|   IBIS model for TI xxx DSP
[IBIS Ver]   5.1
[Disclaimer]   Please be aware that in the absence of a written agreement
|   Texas Instruments(TI) assumes no liability for:
|   (1) The accuracy of the IBIS models provided to your company,
|   however, the IBIS model is compliant to industry standard
|   IQ Level 2a.  Refer to IBIS Quality Section below for
|   for full details.
|   (2) The proper functioning of these Models in your design
|   or for any resulting applications
|   (3) Infringement of patents, copyrights or intellectual
|   property rights resulting from your use of these
|   models.
|   TI provides IBIS Models as a service to our customers and
|   therefore reserves the right to limit distribution of the
|   Models.  The information is subject to change without notice.
[File Name]  sprm812.ibs
[File Rev]   0.1
|   -Initial version
|   -Updated Package model
[Date]   28 July 2022
[Source]   Texas Instruments Incorporated
[Copyright]   Property of Texas Instruments Incorporated.
|   Unauthorized reproduction and/or distribution is strictly.
|   prohibited.
|   This product is protected under copyright law and trade
|   secret law as an unpublished work.
|   Created 2012,(C) Copyright 1999-2012,
|   Texas Instruments Incorporated., All Rights Reserved.
|   These commodities are under the U.S. Government
|   distribution license control. As such,they are not to be
|   re-exported without the prior approval of the U.S.
|   Department of Commerce.
[Notes]
   ADC pins are marked as NC
   Clock pins are marked as NC
   nReset pin marked as NC
   TEMP Sensor pins marked as NC
|   Revision History
|   GERNERAL COMMENT: All IBIS Quality Notes below reflect latest release
|   and version of IBIS File
|   File passes ibischk6.0 with 0 errors and 24 warnings
|   Component AM273
[Component] AM273
[Manufacturer] Texas Instruments
[Package Model] AM273_pkg
[Package]
|   typ   min   max
R_pkg   0.21352   0.10892   0.28767
L_pkg   3.868e-9   1.764e-9   5.903e-9
C_pkg   4.82e-13   3.248e-13   8.016e-13
[Pin]   Signal_name   model_name
M1   VBGAP   POWER
E4   VDD   POWER
E5   VDD   POWER
H4   VDD   POWER
H5   VDD   POWER
L4   VDD   POWER
L5   VDD   POWER
D7   VDD   POWER
M7   VDD   POWER
D9   VDD   POWER
M9   VDD   POWER
H11   VDD   POWER
L11   VDD   POWER
H12   VDD   POWER
L12   VDD   POWER
E11   VDD   POWER
E12   VDD   POWER
K14   VDD_SRAM1   POWER
G3   VDD_SRAM2   POWER
M6   VDD_SRAM3   POWER
F4   VIOIN   POWER
C10   VIOIN   POWER
N10   VIOIN   POWER
F13   VIOIN   POWER
K13   VIOIN   POWER
J4   VIOIN_18   POWER
C8   VIOIN_18   POWER
N8   VIOIN_18   POWER
J12   VIOIN_18   POWER
M2   VIOIN_18ADC   POWER
N2   VIOIN_18CLK   POWER
L13   VNWA   POWER
N7   VPP   POWER
L1   ADC1   NC
P3   ADC2   NC
K2   ADC3   NC
K1   ADC4   NC
J1   ADC5   NC
L2   ADC6   NC
N3   ADC7   NC
J2   ADC8   NC
M3   ADC9   NC
N1   CLKM   NC
P1   CLKP   NC
D2   MSS_EPWMA0   bc1833dv40dcpbfbp18ll_ssdlv
C13   MSS_EPWMA1   bc1833dv40dcpbfbp18ll_ssdlv
D15   MSS_EPWMA_SYNCI   bc1833dv40dcpbfbp18ll_ssdlv
D3   MSS_EPWMB0   bc1833dv40dcpbfbp18ll_ssdlv
D14   MSS_EPWMB1   bc1833dv40dcpbfbp18ll_ssdlv
E1   MSS_EPWMC0   bc1833dv40dcpbfbp18ll_ssdlv
D13   MSS_EPWMC1   bc1833dv40dcpbfbp18ll_ssdlv
F3   MSS_GPIO_0   bc1833dv40dcpbfbp18ll_ssdlv
F2   MSS_GPIO_1   bc1833dv40dcpbfbp18ll_ssdlv
F1   MSS_GPIO_2   bc1833dv40dcpbfbp18ll_ssdlv
E15   MSS_GPIO_7   bc1833dv40dcpbfbp18ll_ssdlv
B4   MSS_GPIO_8   bc1833dv40dcpbfbp18ll_ssdlv
E3   MSS_GPIO_14   bc1833dv40dcpbfbp18ll_ssdlv
E2   MSS_GPIO_28   bc1833dv40dcpbfbp18ll_ssdlv
C14   MSS_GPIO_29   bc1833dv40dcpbfbp18ll_ssdlv
A3   MSS_I2CA_SCL   bc1833dv40dcpbfbp18ll_ssdlv
A4   MSS_I2CA_SDA   bc1833dv40dcpbfbp18ll_ssdlv
B3   MSS_MCANA_RX   bc1833dv40dcpbfbp18ll_ssdlv
C3   MSS_MCANA_TX   bc1833dv40dcpbfbp18ll_ssdlv
M15   MSS_MDIO_CLK   bc1833dv40dcpbfbp18ll_ssdlv
M14   MSS_MDIO_DATA   bc1833dv40dcpbfbp18ll_ssdlv
B14   MSS_MIBSPIB_CLK   bc1833dv40dcpbfbp18ll_ssdlv
B15   MSS_MIBSPIB_CS0   bc1833dv40dcpbfbp18ll_ssdlv
C15   MSS_MIBSPIB_CS1   bc1833dv40dcpbfbp18ll_ssdlv
A14   MSS_MIBSPIB_MISO   bc1833dv40dcpbfbp18ll_ssdlv
B13   MSS_MIBSPIB_MOSI   bc1833dv40dcpbfbp18ll_ssdlv
B2   MSS_QSPI_0   bc1833dv40dcpbfbp18ll_ssdlv
A2   MSS_QSPI_1   bc1833dv40dcpbfbp18ll_ssdlv
C2   MSS_QSPI_2   bc1833dv40dcpbfbp18ll_ssdlv
B1   MSS_QSPI_3   bc1833dv40dcpbfbp18ll_ssdlv
D1   MSS_QSPI_CLK   bc1833dv40dcpbfbp18ll_ssdlv
C1   MSS_QSPI_CS   bc1833dv40dcpbfbp18ll_ssdlv
K15   MSS_RGMII_RCLK   bc1833dv40dcpbfbp18ll_ssdlv
G13   MSS_RGMII_RCTL   bc1833dv40dcpbfbp18ll_ssdlv
M13   MSS_RGMII_RD0   bc1833dv40dcpbfbp18ll_ssdlv
L15   MSS_RGMII_RD1   bc1833dv40dcpbfbp18ll_ssdlv
L14   MSS_RGMII_RD2   bc1833dv40dcpbfbp18ll_ssdlv
J13   MSS_RGMII_RD3   bc1833dv40dcpbfbp18ll_ssdlv
H15   MSS_RGMII_TCLK   bc1833dv40dcpbfbp18ll_ssdlv
G15   MSS_RGMII_TCTL   bc1833dv40dcpbfbp18ll_ssdlv
J14   MSS_RGMII_TD0   bc1833dv40dcpbfbp18ll_ssdlv
J15   MSS_RGMII_TD1   bc1833dv40dcpbfbp18ll_ssdlv
H13   MSS_RGMII_TD2   bc1833dv40dcpbfbp18ll_ssdlv
H14   MSS_RGMII_TD3   bc1833dv40dcpbfbp18ll_ssdlv
R3   MSS_UARTA_RX   bc1833dv40dcpbfbp18ll_ssdlh
R4   MSS_UARTA_TX   bc1833dv40dcpbfbp18ll_ssdlh
P4   MSS_UARTB_TX   bc1833dv40dcpbfbp18ll_ssdlh
H2   NERROR_IN   bc1833dv40dcpbfbp18ll_od_fs_ssdlv
H1   NERROR_OUT   bc1833dv40dcpbfbp18ll_od_fs_ssdlv
J3   NRESET   NC
R2   OSC_CLK_OUT_AUDIO   NC
E14   RCSS_ECAPA_CAPIN_PWMO   bc1833dv40dcpbfbp18ll_ssdlv
R14   RCSS_GPIO_39   bc1833dv40dcpbfbp18ll_ssdlv
R13   RCSS_I2CA_SCL   bc1833dv40dcpbfbp18ll_ssdlv
P13   RCSS_I2CA_SDA   bc1833dv40dcpbfbp18ll_ssdlv
B12   RCSS_MCASPA_ACLKR   bc1833dv40dcpbfbp18ll_ssdlh
A12   RCSS_MCASPA_ACLKX   bc1833dv40dcpbfbp18ll_ssdlh
A13   RCSS_MCASPA_AHCLKX   bc1833dv40dcpbfbp18ll_ssdlh
B11   RCSS_MCASPA_DAT0   bc1833dv40dcpbfbp18ll_ssdlh
C11   RCSS_MCASPA_DAT1   bc1833dv40dcpbfbp18ll_ssdlh
B7   RCSS_MCASPA_DAT2   bc1833dv40dcpbfbp18ll_ssdlh
C7   RCSS_MCASPA_DAT3   bc1833dv40dcpbfbp18ll_ssdlh
B6   RCSS_MCASPA_DAT4   bc1833dv40dcpbfbp18ll_ssdlh
A6   RCSS_MCASPA_DAT5   bc1833dv40dcpbfbp18ll_ssdlh
B5   RCSS_MCASPA_DAT6   bc1833dv40dcpbfbp18ll_ssdlh
A5   RCSS_MCASPA_DAT7   bc1833dv40dcpbfbp18ll_ssdlh
B10   RCSS_MCASPA_DAT8   bc1833dv40dcpbfbp18ll_ssdlh
A10   RCSS_MCASPA_DAT9   bc1833dv40dcpbfbp18ll_ssdlh
A9   RCSS_MCASPA_DAT10   bc1833dv40dcpbfbp18ll_ssdlh
C9   RCSS_MCASPA_DAT11   bc1833dv40dcpbfbp18ll_ssdlh
B9   RCSS_MCASPA_DAT12   bc1833dv40dcpbfbp18ll_ssdlh
A8   RCSS_MCASPA_DAT13   bc1833dv40dcpbfbp18ll_ssdlh
B8   RCSS_MCASPA_DAT14   bc1833dv40dcpbfbp18ll_ssdlh
A7   RCSS_MCASPA_DAT15   bc1833dv40dcpbfbp18ll_ssdlh
A11   RCSS_MCASPA_FSR   bc1833dv40dcpbfbp18ll_ssdlh
C12   RCSS_MCASPA_FSX   bc1833dv40dcpbfbp18ll_ssdlh
P7   RCSS_MCASPB_ACLKR   bc1833dv40dcpbfbp18ll_ssdlh
R8   RCSS_MCASPB_ACLKX   bc1833dv40dcpbfbp18ll_ssdlh
R7   RCSS_MCASPB_AHCLKX   bc1833dv40dcpbfbp18ll_ssdlh
R6   RCSS_MCASPB_DAT0   bc1833dv40dcpbfbp18ll_ssdlh
N5   RCSS_MCASPB_DAT1   bc1833dv40dcpbfbp18ll_ssdlh
P5   RCSS_MCASPB_DAT2   bc1833dv40dcpbfbp18ll_ssdlh
R5   RCSS_MCASPB_DAT3   bc1833dv40dcpbfbp18ll_ssdlh
N4   RCSS_MCASPB_DAT4   bc1833dv40dcpbfbp18ll_ssdlh
N6   RCSS_MCASPB_DAT5   bc1833dv40dcpbfbp18ll_ssdlh
P6   RCSS_MCASPB_FSR   bc1833dv40dcpbfbp18ll_ssdlh
P8   RCSS_MCASPB_FSX   bc1833dv40dcpbfbp18ll_ssdlh
R10   RCSS_MCASPC_ACLKR   bc1833dv40dcpbfbp18ll_ssdlh
R9   RCSS_MCASPC_ACLKX   bc1833dv40dcpbfbp18ll_ssdlh
P9   RCSS_MCASPC_AHCLKX   bc1833dv40dcpbfbp18ll_ssdlh
R11   RCSS_MCASPC_DAT0   bc1833dv40dcpbfbp18ll_ssdlh
P11   RCSS_MCASPC_DAT1   bc1833dv40dcpbfbp18ll_ssdlh
N11   RCSS_MCASPC_DAT2   bc1833dv40dcpbfbp18ll_ssdlh
R12   RCSS_MCASPC_DAT3   bc1833dv40dcpbfbp18ll_ssdlh
P12   RCSS_MCASPC_DAT4   bc1833dv40dcpbfbp18ll_ssdlh
N12   RCSS_MCASPC_DAT5   bc1833dv40dcpbfbp18ll_ssdlh
P10   RCSS_MCASPC_FSR   bc1833dv40dcpbfbp18ll_ssdlh
N9   RCSS_MCASPC_FSX   bc1833dv40dcpbfbp18ll_ssdlh
P15   RCSS_MIBSPIA_CLK   bc1833dv40dcpbfbp18ll_ssdlv
P14   RCSS_MIBSPIA_CS0   bc1833dv40dcpbfbp18ll_ssdlv
N13   RCSS_MIBSPIA_CS1   bc1833dv40dcpbfbp18ll_ssdlv
N14   RCSS_MIBSPIA_MISO   bc1833dv40dcpbfbp18ll_ssdlv
N15   RCSS_MIBSPIA_MOSI   bc1833dv40dcpbfbp18ll_ssdlv
E13   RCSS_UARTA_CTS   bc1833dv40dcpbfbp18ll_ssdlv
F15   RCSS_UARTA_RTS   bc1833dv40dcpbfbp18ll_ssdlv
G14   RCSS_UARTA_RX   bc1833dv40dcpbfbp18ll_ssdlv
F14   RCSS_UARTA_TX   bc1833dv40dcpbfbp18ll_ssdlv
D4   TCK   bc1833dv40dcpbfbp18ll_ssdlh
C5   TDI   bc1833dv40dcpbfbp18ll_ssdlh
C6   TDO   bc1833dv40dcpbfbp18ll_ssdlh
L3   TEMP_SENSOR_1   NC
K3   TEMP_SENSOR_2   NC
C4   TMS   bc1833dv40dcpbfbp18ll_ssdlh
H3   WARM_RESET   bc1833dv40dcpbfbp18ll_od_fs_ssdlv
G1   XREF_CLK0   NC
G2   XREF_CLK1   NC
R1   VSS   GND
P2   VSS   GND
A1   VSS   GND
D5   VSS   GND
D6   VSS   GND
G4   VSS   GND
K4   VSS   GND
M8   VSS   GND
D11   VSS   GND
D12   VSS   GND
F5   VSS   GND
G5   VSS   GND
K5   VSS   GND
J5   VSS   GND
E6   VSS   GND
F6   VSS   GND
H6   VSS   GND
G6   VSS   GND
K6   VSS   GND
J6   VSS   GND
L6   VSS   GND
E7   VSS   GND
E8   VSS   GND
D8   VSS   GND
F7   VSS   GND
F8   VSS   GND
H7   VSS   GND
G7   VSS   GND
H8   VSS   GND
G8   VSS   GND
K7   VSS   GND
J7   VSS   GND
K8   VSS   GND
J8   VSS   GND
L7   VSS   GND
L8   VSS   GND
E9   VSS   GND
E10   VSS   GND
D10   VSS   GND
F9   VSS   GND
F10   VSS   GND
H9   VSS   GND
G9   VSS   GND
H10   VSS   GND
G10   VSS   GND
K9   VSS   GND
J9   VSS   GND
K10   VSS   GND
J10   VSS   GND
L9   VSS   GND
L10   VSS   GND
M10   VSS   GND
F11   VSS   GND
G11   VSS   GND
K11   VSS   GND
J11   VSS   GND
M11   VSS   GND
F12   VSS   GND
G12   VSS   GND
M12   VSS   GND
M5   VSS   GND
M4   VSS   GND
K12   VSS   GND
R15   VSS   GND
A15   VSS   GND
|   BC1833DV40DCPBFBP18LL_SSDLH
[Model Selector] bc1833dv40dcpbfbp18ll_ssdlh
|SC1 IS A SLEW RATE CONTROL PIN
|5% SUPPLY VARIATION MODES WITH 1.8V NOM SUPPLY
BC40D_H_PUPDOFF_5P_SC1_1P8  Cell operated at 1.8(nom)
|BC40D_H_PUPDOFF_5P_SC1_1P8; BUFFER WITH WEAK PULUP/PULLDOWN OFF AT 5% SUPPLY
|VARIATION WITH SC1=1 MEANING SLOW MODE OF OPERATION
BC40D_H_PD_ON_5P_!SC1_1P8  Cell operated at 1.8(nom)
|BC40D_H_PD_ON_5P_!SC1_1P8; BUFFER WITH WEAK_PULLDOWN_ON AT 5% SUPPLY
|VARIATION WITH SC1=0 MEANING FAST MODE OF OPERATION
BC40D_H_PD_ON_5P_SC1_1P8  Cell operated at 1.8(nom)
|BC40D_H_PD_ON_5P_SC1_1P8; BUFFER WITH WEAK_PULLDOWN_ON AT 5% SUPPLY
|VARIATION WITH SC1=1 MEANING SLOW MODE OF OPERATION
BC40D_H_PU_ON_5P_!SC1_1P8  Cell operated at 1.8(nom)
|BC40D_H_PU_ON_5P_!SC1_1P8; BUFFER WITH WEAK_PULLUP_ON AT 5% SUPPLY
|VARIATION WITH SC1=0 MEANING FAST MODE OF OPERATION
BC40D_H_PUPDOFF_5P_!SC1_1P8  Cell operated at 1.8(nom)
|BC40D_H_PUPDOFF_5P_!SC1_1P8; BUFFER WITH WEAK PULUP/PULLDOWN OFF AT 5% SUPPLY
|VARIATION WITH SC1=0 MEANING FAST MODE OF OPERATION
BC40D_H_PU_ON_5P_SC1_1P8  Cell operated at 1.8(nom)
|BC40D_H_PU_ON_5P_SC1_1P8; BUFFER WITH WEAK_PULLUP_ON AT 5% SUPPLY
|VARIATION WITH SC1=1 MEANING SLOW MODE OF OPERATION
|5% SUPPLY VARIATION MODES WITH 3.3V NOM SUPPLY
BC40D_H_PUPDOFF_5P_SC1_3P3  Cell operated at 3.3(nom)
|BC40D_H_PUPDOFF_5P_SC1_3P3; BUFFER WITH WEAK PULUP/PULLDOWN OFF AT 5% SUPPLY
|VARIATION WITH SC1=1 MEANING SLOW MODE OF OPERATION
BC40D_H_PD_ON_5P_!SC1_3P3  Cell operated at 3.3(nom)
|BC40D_H_PD_ON_5P_!SC1_3P3; BUFFER WITH WEAK_PULLDOWN_ON AT 5% SUPPLY
|VARIATION WITH SC1=0 MEANING FAST MODE OF OPERATION
BC40D_H_PD_ON_5P_SC1_3P3  Cell operated at 3.3(nom)
|BC40D_H_PD_ON_5P_SC1_3P3; BUFFER WITH WEAK_PULLDOWN_ON AT 5% SUPPLY
|VARIATION WITH SC1=1 MEANING SLOW MODE OF OPERATION
BC40D_H_PU_ON_5P_!SC1_3P3  Cell operated at 3.3(nom)
|BC40D_H_PU_ON_5P_!SC1_3P3; BUFFER WITH WEAK_PULLUP_ON AT 5% SUPPLY
|VARIATION WITH SC1=0 MEANING FAST MODE OF OPERATION
BC40D_H_PUPDOFF_5P_!SC1_3P3  Cell operated at 3.3(nom)
|BC40D_H_PUPDOFF_5P_!SC1_3P3; BUFFER WITH WEAK PULUP/PULLDOWN OFF AT 5% SUPPLY
|VARIATION WITH SC1=0 MEANING FAST MODE OF OPERATION
BC40D_H_PU_ON_5P_SC1_3P3  Cell operated at 3.3(nom)
|BC40D_H_PU_ON_5P_SC1_3P3; BUFFER WITH WEAK_PULLUP_ON AT 5% SUPPLY
|VARIATION WITH SC1=1 MEANING SLOW MODE OF OPERATION
| 10% SUPPLY VARIATION MODES WITH 1.8V NOM SUPPLY
BC40D_H_PUPDOFF_10P_SC1_1P8  Cell operated at 1.8(nom)
|BC40D_H_PUPDOFF_10P_SC1_1P8; BUFFER WITH WEAK PULUP/PULLDOWN OFF AT 10% SUPPLY
|VARIATION WITH SC1=1 MEANING SLOW MODE OF OPERATION
BC40D_H_PD_ON_10P_!SC1_1P8  Cell operated at 1.8(nom)
|BC40D_H_PD_ON_10P_!SC1_1P8; BUFFER WITH WEAK_PULLDOWN_ON AT 10% SUPPLY
|VARIATION WITH SC1=0 MEANING FAST MODE OF OPERATION
BC40D_H_PD_ON_10P_SC1_1P8  Cell operated at 1.8(nom)
|BC40D_H_PD_ON_10P_SC1_1P8; BUFFER WITH WEAK_PULLDOWN_ON AT 10% SUPPLY
|VARIATION WITH SC1=1 MEANING SLOW MODE OF OPERATION
BC40D_H_PU_ON_10P_!SC1_1P8  Cell operated at 1.8(nom)
|BC40D_H_PU_ON_10P_!SC1_1P8; BUFFER WITH WEAK_PULLUP_ON AT 10% SUPPLY
|VARIATION WITH SC1=0 MEANING FAST MODE OF OPERATION
BC40D_H_PUPDOFF_10P_!SC1_1P8  Cell operated at 1.8(nom)
|BC40D_H_PUPDOFF_10P_!SC1_1P8; BUFFER WITH WEAK PULUP/PULLDOWN OFF AT 10% SUPPLY
|VARIATION WITH SC1=0 MEANING FAST MODE OF OPERATION
BC40D_H_PU_ON_10P_SC1_1P8  Cell operated at 1.8(nom)
|BC40D_H_PU_ON_10P_SC1_1P8; BUFFER WITH WEAK_PULLUP_ON AT 10% SUPPLY
|VARIATION WITH SC1=1 MEANING SLOW MODE OF OPERATION
| 10% SUPPLY VARIATION MODES WITH 3.3V NOM SUPPLY
BC40D_H_PUPDOFF_10P_SC1_3P3  Cell operated at 3.3(nom)
|BC40D_H_PUPDOFF_10P_SC1_3P3; BUFFER WITH WEAK PULUP/PULLDOWN OFF AT 10% SUPPLY
|VARIATION WITH SC1=1 MEANING SLOW MODE OF OPERATION
BC40D_H_PD_ON_10P_!SC1_3P3  Cell operated at 3.3(nom)
|BC40D_H_PD_ON_10P_!SC1_3P3; BUFFER WITH WEAK_PULLDOWN_ON 10% SUPPLY
|VARIATION WITH SC1=0 MEANING FAST MODE OF OPERATION
BC40D_H_PD_ON_10P_SC1_3P3  Cell operated at 3.3(nom)
|BC40D_H_PD_ON_10P_SC1_3P3; BUFFER WITH WEAK_PULLDOWN_ON AT 10% SUPPLY
|VARIATION WITH SC1=1 MEANING SLOW MODE OF OPERATION
BC40D_H_PU_ON_10P_!SC1_3P3  Cell operated at 3.3(nom)
|BC40D_H_PU_ON_10P_!SC1_3P3; BUFFER WITH WEAK_PULLUP_ON AT 10% SUPPLY
|VARIATION WITH SC1=0 MEANING FAST MODE OF OPERATION
BC40D_H_PUPDOFF_10P_!SC1_3P3  Cell operated at 3.3(nom)
|BC40D_H_PUPDOFF_10P_!SC1_3P3; BUFFER WITH WEAK PULUP/PULLDOWN OFF AT 10% SUPPLY
|VARIATION WITH SC1=0 MEANING FAST MODE OF OPERATION
BC40D_H_PU_ON_10P_SC1_3P3  Cell operated at 3.3(nom)
|BC40D_H_PU_ON_10P_SC1_3P3; BUFFER WITH WEAK_PULLUP_ON AT 10% SUPPLY
|VARIATION WITH SC1=1 MEANING SLOW MODE OF OPERATION
|   BC1833DV40DCPBFBP18LL_SSDLV
[Model Selector] bc1833dv40dcpbfbp18ll_ssdlv
|SC1 IS A SLEW RATE CONTROL PIN
|5% SUPPLY VARIATION MODES WITH 1.8V NOM SUPPLY
BC40D_V_PUPDOFF_5P_SC1_1P8  Cell operated at 1.8(nom)
|BC40D_V_PUPDOFF_5P_SC1_1P8; BUFFER WITH WEAK PULUP/PULLDOWN OFF AT 5% SUPPLY
|VARIATION WITH SC1=1 MEANING SLOW MODE OF OPERATION
BC40D_V_PD_ON_5P_!SC1_1P8  Cell operated at 1.8(nom)
|BC40D_V_PD_ON_5P_!SC1_1P8; BUFFER WITH WEAK_PULLDOWN_ON AT 5% SUPPLY
|VARIATION WITH SC1=0 MEANING FAST MODE OF OPERATION
BC40D_V_PD_ON_5P_SC1_1P8  Cell operated at 1.8(nom)
|BC40D_V_PD_ON_5P_SC1_1P8; BUFFER WITH WEAK_PULLDOWN_ON AT 5% SUPPLY
|VARIATION WITH SC1=1 MEANING SLOW MODE OF OPERATION
BC40D_V_PU_ON_5P_!SC1_1P8  Cell operated at 1.8(nom)
|BC40D_V_PU_ON_5P_!SC1_1P8; BUFFER WITH WEAK_PULLUP_ON AT 5% SUPPLY
|VARIATION WITH SC1=0 MEANING FAST MODE OF OPERATION
BC40D_V_PUPDOFF_5P_!SC1_1P8  Cell operated at 1.8(nom)
|BC40D_V_PUPDOFF_5P_!SC1_1P8; BUFFER WITH WEAK PULUP/PULLDOWN OFF AT 5% SUPPLY
|VARIATION WITH SC1=0 MEANING FAST MODE OF OPERATION
BC40D_V_PU_ON_5P_SC1_1P8  Cell operated at 1.8(nom)
|BC40D_V_PU_ON_5P_SC1_1P8; BUFFER WITH WEAK_PULLUP_ON AT 5% SUPPLY
|VARIATION WITH SC1=1 MEANING SLOW MODE OF OPERATION
|5% SUPPLY VARIATION MODES WITH 3.3V NOM SUPPLY
BC40D_V_PUPDOFF_5P_SC1_3P3  Cell operated at 3.3(nom)
|BC40D_V_PUPDOFF_5P_SC1_3P3; BUFFER WITH WEAK PULUP/PULLDOWN OFF AT 5% SUPPLY
|VARIATION WITH SC1=1 MEANING SLOW MODE OF OPERATION
BC40D_V_PD_ON_5P_!SC1_3P3  Cell operated at 3.3(nom)
|BC40D_V_PD_ON_5P_!SC1_3P3; BUFFER WITH WEAK_PULLDOWN_ON AT 5% SUPPLY
|VARIATION WITH SC1=0 MEANING FAST MODE OF OPERATION
BC40D_V_PD_ON_5P_SC1_3P3  Cell operated at 3.3(nom)
|BC40D_V_PD_ON_5P_SC1_3P3; BUFFER WITH WEAK_PULLDOWN_ON AT 5% SUPPLY
|VARIATION WITH SC1=1 MEANING SLOW MODE OF OPERATION
BC40D_V_PU_ON_5P_!SC1_3P3  Cell operated at 3.3(nom)
|BC40D_V_PU_ON_5P_!SC1_3P3; BUFFER WITH WEAK_PULLUP_ON AT 5% SUPPLY
|VARIATION WITH SC1=0 MEANING FAST MODE OF OPERATION
BC40D_V_PUPDOFF_5P_!SC1_3P3  Cell operated at 3.3(nom)
|BC40D_V_PUPDOFF_5P_!SC1_3P3; BUFFER WITH WEAK PULUP/PULLDOWN OFF AT 5% SUPPLY
|VARIATION WITH SC1=0 MEANING FAST MODE OF OPERATION
BC40D_V_PU_ON_5P_SC1_3P3  Cell operated at 3.3(nom)
|BC40D_V_PU_ON_5P_SC1_3P3; BUFFER WITH WEAK_PULLUP_ON AT 5% SUPPLY
|VARIATION WITH SC1=1 MEANING SLOW MODE OF OPERATION
| 10% SUPPLY VARIATION MODES WITH 1.8V NOM SUPPLY
BC40D_V_PUPDOFF_10P_SC1_1P8  Cell operated at 1.8(nom)
|BC40D_V_PUPDOFF_10P_SC1_1P8; BUFFER WITH WEAK PULUP/PULLDOWN OFF AT 10% SUPPLY
|VARIATION WITH SC1=1 MEANING SLOW MODE OF OPERATION
BC40D_V_PD_ON_10P_!SC1_1P8  Cell operated at 1.8(nom)
|BC40D_V_PD_ON_10P_!SC1_1P8; BUFFER WITH WEAK_PULLDOWN_ON AT 10% SUPPLY
|VARIATION WITH SC1=0 MEANING FAST MODE OF OPERATION
BC40D_V_PD_ON_10P_SC1_1P8  Cell operated at 1.8(nom)
|BC40D_V_PD_ON_10P_SC1_1P8; BUFFER WITH WEAK_PULLDOWN_ON AT 10% SUPPLY
|VARIATION WITH SC1=1 MEANING SLOW MODE OF OPERATION
BC40D_V_PU_ON_10P_!SC1_1P8  Cell operated at 1.8(nom)
|BC40D_V_PU_ON_10P_!SC1_1P8; BUFFER WITH WEAK_PULLUP_ON AT 10% SUPPLY
|VARIATION WITH SC1=0 MEANING FAST MODE OF OPERATION
BC40D_V_PUPDOFF_10P_!SC1_1P8  Cell operated at 1.8(nom)
|BC40D_V_PUPDOFF_10P_!SC1_1P8; BUFFER WITH WEAK PULUP/PULLDOWN OFF AT 10% SUPPLY
|VARIATION WITH SC1=0 MEANING FAST MODE OF OPERATION
BC40D_V_PU_ON_10P_SC1_1P8  Cell operated at 1.8(nom)
|BC40D_V_PU_ON_10P_SC1_1P8; BUFFER WITH WEAK_PULLUP_ON AT 10% SUPPLY
|VARIATION WITH SC1=1 MEANING SLOW MODE OF OPERATION
| 10% SUPPLY VARIATION MODES WITH 3.3V NOM SUPPLY
BC40D_V_PUPDOFF_10P_SC1_3P3  Cell operated at 3.3(nom)
|BC40D_V_PUPDOFF_10P_SC1_3P3; BUFFER WITH WEAK PULUP/PULLDOWN OFF AT 10% SUPPLY
|VARIATION WITH SC1=1 MEANING SLOW MODE OF OPERATION
BC40D_V_PD_ON_10P_!SC1_3P3  Cell operated at 3.3(nom)
|BC40D_V_PD_ON_10P_!SC1_3P3; BUFFER WITH WEAK_PULLDOWN_ON 10% SUPPLY
|VARIATION WITH SC1=0 MEANING FAST MODE OF OPERATION
BC40D_V_PD_ON_10P_SC1_3P3  Cell operated at 3.3(nom)
|BC40D_V_PD_ON_10P_SC1_3P3; BUFFER WITH WEAK_PULLDOWN_ON AT 10% SUPPLY
|VARIATION WITH SC1=1 MEANING SLOW MODE OF OPERATION
BC40D_V_PU_ON_10P_!SC1_3P3  Cell operated at 3.3(nom)
|BC40D_V_PU_ON_10P_!SC1_3P3; BUFFER WITH WEAK_PULLUP_ON AT 10% SUPPLY
|VARIATION WITH SC1=0 MEANING FAST MODE OF OPERATION
BC40D_V_PUPDOFF_10P_!SC1_3P3  Cell operated at 3.3(nom)
|BC40D_V_PUPDOFF_10P_!SC1_3P3; BUFFER WITH WEAK PULUP/PULLDOWN OFF AT 10% SUPPLY
|VARIATION WITH SC1=0 MEANING FAST MODE OF OPERATION
BC40D_V_PU_ON_10P_SC1_3P3  Cell operated at 3.3(nom)
|BC40D_V_PU_ON_10P_SC1_3P3; BUFFER WITH WEAK_PULLUP_ON AT 10% SUPPLY
|VARIATION WITH SC1=1 MEANING SLOW MODE OF OPERATION
|   BC1833DV40DCPBFBP18LL_OD_FS_SSDLV
[Model Selector] bc1833dv40dcpbfbp18ll_od_fs_ssdlv
|SC1 IS A SLEW RATE CONTROL PIN
|5% SUPPLY VARIATION MODES WITH 1.8V NOM SUPPLY
BC40D_V_PUPDOFF_5P_SC1_1P8  Cell operated at 1.8(nom)
|BC40D_V_PUPDOFF_5P_SC1_1P8; BUFFER WITH WEAK PULUP/PULLDOWN OFF AT 5% SUPPLY
|VARIATION WITH SC1=1 MEANING SLOW MODE OF OPERATION
BC40D_V_PD_ON_5P_!SC1_1P8  Cell operated at 1.8(nom)
|BC40D_V_PD_ON_5P_!SC1_1P8; BUFFER WITH WEAK_PULLDOWN_ON AT 5% SUPPLY
|VARIATION WITH SC1=0 MEANING FAST MODE OF OPERATION
BC40D_V_PD_ON_5P_SC1_1P8  Cell operated at 1.8(nom)
|BC40D_V_PD_ON_5P_SC1_1P8; BUFFER WITH WEAK_PULLDOWN_ON AT 5% SUPPLY
|VARIATION WITH SC1=1 MEANING SLOW MODE OF OPERATION
BC40D_V_PU_ON_5P_!SC1_1P8  Cell operated at 1.8(nom)
|BC40D_V_PU_ON_5P_!SC1_1P8; BUFFER WITH WEAK_PULLUP_ON AT 5% SUPPLY
|VARIATION WITH SC1=0 MEANING FAST MODE OF OPERATION
BC40D_V_PUPDOFF_5P_!SC1_1P8  Cell operated at 1.8(nom)
|BC40D_V_PUPDOFF_5P_!SC1_1P8; BUFFER WITH WEAK PULUP/PULLDOWN OFF AT 5% SUPPLY
|VARIATION WITH SC1=0 MEANING FAST MODE OF OPERATION
BC40D_V_PU_ON_5P_SC1_1P8  Cell operated at 1.8(nom)
|BC40D_V_PU_ON_5P_SC1_1P8; BUFFER WITH WEAK_PULLUP_ON AT 5% SUPPLY
|VARIATION WITH SC1=1 MEANING SLOW MODE OF OPERATION
|5% SUPPLY VARIATION MODES WITH 3.3V NOM SUPPLY
BC40D_V_PUPDOFF_5P_SC1_3P3  Cell operated at 3.3(nom)
|BC40D_V_PUPDOFF_5P_SC1_3P3; BUFFER WITH WEAK PULUP/PULLDOWN OFF AT 5% SUPPLY
|VARIATION WITH SC1=1 MEANING SLOW MODE OF OPERATION
BC40D_V_PD_ON_5P_!SC1_3P3  Cell operated at 3.3(nom)
|BC40D_V_PD_ON_5P_!SC1_3P3; BUFFER WITH WEAK_PULLDOWN_ON AT 5% SUPPLY
|VARIATION WITH SC1=0 MEANING FAST MODE OF OPERATION
BC40D_V_PD_ON_5P_SC1_3P3  Cell operated at 3.3(nom)
|BC40D_V_PD_ON_5P_SC1_3P3; BUFFER WITH WEAK_PULLDOWN_ON AT 5% SUPPLY
|VARIATION WITH SC1=1 MEANING SLOW MODE OF OPERATION
BC40D_V_PU_ON_5P_!SC1_3P3  Cell operated at 3.3(nom)
|BC40D_V_PU_ON_5P_!SC1_3P3; BUFFER WITH WEAK_PULLUP_ON AT 5% SUPPLY
|VARIATION WITH SC1=0 MEANING FAST MODE OF OPERATION
BC40D_V_PUPDOFF_5P_!SC1_3P3  Cell operated at 3.3(nom)
|BC40D_V_PUPDOFF_5P_!SC1_3P3; BUFFER WITH WEAK PULUP/PULLDOWN OFF AT 5% SUPPLY
|VARIATION WITH SC1=0 MEANING FAST MODE OF OPERATION
BC40D_V_PU_ON_5P_SC1_3P3  Cell operated at 3.3(nom)
|BC40D_V_PU_ON_5P_SC1_3P3; BUFFER WITH WEAK_PULLUP_ON AT 5% SUPPLY
|VARIATION WITH SC1=1 MEANING SLOW MODE OF OPERATION
| 10% SUPPLY VARIATION MODES WITH 1.8V NOM SUPPLY
BC40D_V_PUPDOFF_10P_SC1_1P8  Cell operated at 1.8(nom)
|BC40D_V_PUPDOFF_10P_SC1_1P8; BUFFER WITH WEAK PULUP/PULLDOWN OFF AT 10% SUPPLY
|VARIATION WITH SC1=1 MEANING SLOW MODE OF OPERATION
BC40D_V_PD_ON_10P_!SC1_1P8  Cell operated at 1.8(nom)
|BC40D_V_PD_ON_10P_!SC1_1P8; BUFFER WITH WEAK_PULLDOWN_ON AT 10% SUPPLY
|VARIATION WITH SC1=0 MEANING FAST MODE OF OPERATION
BC40D_V_PD_ON_10P_SC1_1P8  Cell operated at 1.8(nom)
|BC40D_V_PD_ON_10P_SC1_1P8; BUFFER WITH WEAK_PULLDOWN_ON AT 10% SUPPLY
|VARIATION WITH SC1=1 MEANING SLOW MODE OF OPERATION
BC40D_V_PU_ON_10P_!SC1_1P8  Cell operated at 1.8(nom)
|BC40D_V_PU_ON_10P_!SC1_1P8; BUFFER WITH WEAK_PULLUP_ON AT 10% SUPPLY
|VARIATION WITH SC1=0 MEANING FAST MODE OF OPERATION
BC40D_V_PUPDOFF_10P_!SC1_1P8  Cell operated at 1.8(nom)
|BC40D_V_PUPDOFF_10P_!SC1_1P8; BUFFER WITH WEAK PULUP/PULLDOWN OFF AT 10% SUPPLY
|VARIATION WITH SC1=0 MEANING FAST MODE OF OPERATION
BC40D_V_PU_ON_10P_SC1_1P8  Cell operated at 1.8(nom)
|BC40D_V_PU_ON_10P_SC1_1P8; BUFFER WITH WEAK_PULLUP_ON AT 10% SUPPLY
|VARIATION WITH SC1=1 MEANING SLOW MODE OF OPERATION
| 10% SUPPLY VARIATION MODES WITH 3.3V NOM SUPPLY
BC40D_V_PUPDOFF_10P_SC1_3P3  Cell operated at 3.3(nom)
|BC40D_V_PUPDOFF_10P_SC1_3P3; BUFFER WITH WEAK PULUP/PULLDOWN OFF AT 10% SUPPLY
|VARIATION WITH SC1=1 MEANING SLOW MODE OF OPERATION
BC40D_V_PD_ON_10P_!SC1_3P3  Cell operated at 3.3(nom)
|BC40D_V_PD_ON_10P_!SC1_3P3; BUFFER WITH WEAK_PULLDOWN_ON 10% SUPPLY
|VARIATION WITH SC1=0 MEANING FAST MODE OF OPERATION
BC40D_V_PD_ON_10P_SC1_3P3  Cell operated at 3.3(nom)
|BC40D_V_PD_ON_10P_SC1_3P3; BUFFER WITH WEAK_PULLDOWN_ON AT 10% SUPPLY
|VARIATION WITH SC1=1 MEANING SLOW MODE OF OPERATION
BC40D_V_PU_ON_10P_!SC1_3P3  Cell operated at 3.3(nom)
|BC40D_V_PU_ON_10P_!SC1_3P3; BUFFER WITH WEAK_PULLUP_ON AT 10% SUPPLY
|VARIATION WITH SC1=0 MEANING FAST MODE OF OPERATION
BC40D_V_PUPDOFF_10P_!SC1_3P3  Cell operated at 3.3(nom)
|BC40D_V_PUPDOFF_10P_!SC1_3P3; BUFFER WITH WEAK PULUP/PULLDOWN OFF AT 10% SUPPLY
|VARIATION WITH SC1=0 MEANING FAST MODE OF OPERATION
BC40D_V_PU_ON_10P_SC1_3P3  Cell operated at 3.3(nom)
|   Package Model
[Define Package Model]   AM273_pkg
[Manufacturer]   name 1
[OEM]   name 2
[Description]   138-pin Package
|[Number of Sections]   1
[Number of Pins]   138
[Pin Numbers]
|[Pin Name]  Net Number   Net Name   Net's All Pins
M1   | 1   VBGAP   M1
E4   | 2   VDD   E4
   |E5
   |H4
   |H5
   |L4
   |L5
   |D7
   |M7
   |D9
   |M9
   |H11
   |L11
   |H12
   |L12
   |E11
   |E12
K14   | 3   VDD_SRAM1   K14
G3   | 4   VDD_SRAM2   G3
M6   | 5   VDD_SRAM3   M6
F4   | 6   VIOIN   F4
   |C10
   |N10
   |F13
   |K13
J4   | 7   VIOIN_18   J4
   |C8
   |N8
   |J12
M2   | 8   VIOIN_18ADC   M2
N2   | 9   VIOIN_18CLK   N2
L13   | 10   VNWA   L13
N7   | 11   VPP   N7
L1   | 12   ADC1   L1
P3   | 13   ADC2   P3
K2   | 14   ADC3   K2
K1   | 15   ADC4   K1
J1   | 16   ADC5   J1
L2   | 17   ADC6   L2
N3   | 18   ADC7   N3
J2   | 19   ADC8   J2
M3   | 20   ADC9   M3
N1   | 21   CLKM   N1
P1   | 22   CLKP   P1
D2   | 23   MSS_EPWMA0   D2
C13   | 24   MSS_EPWMA1   C13
D15   | 25   MSS_EPWMA_SYNCI   D15
D3   | 26   MSS_EPWMB0   D3
D14   | 27   MSS_EPWMB1   D14
E1   | 28   MSS_EPWMC0   E1
D13   | 29   MSS_EPWMC1   D13
F3   | 30   MSS_GPIO_0   F3
F2   | 31   MSS_GPIO_1   F2
F1   | 32   MSS_GPIO_2   F1
E15   | 33   MSS_GPIO_7   E15
B4   | 34   MSS_GPIO_8   B4
E3   | 35   MSS_GPIO_14   E3
E2   | 36   MSS_GPIO_28   E2
C14   | 37   MSS_GPIO_29   C14
A3   | 38   MSS_I2CA_SCL   A3
A4   | 39   MSS_I2CA_SDA   A4
B3   | 40   MSS_MCANA_RX   B3
C3   | 41   MSS_MCANA_TX   C3
M15   | 42   MSS_MDIO_CLK   M15
M14   | 43   MSS_MDIO_DATA   M14
B14   | 44   MSS_MIBSPIB_CLK   B14
B15   | 45   MSS_MIBSPIB_CS0   B15
C15   | 46   MSS_MIBSPIB_CS1   C15
A14   | 47   MSS_MIBSPIB_MISO   A14
B13   | 48   MSS_MIBSPIB_MOSI   B13
B2   | 49   MSS_QSPI_0   B2
A2   | 50   MSS_QSPI_1   A2
C2   | 51   MSS_QSPI_2   C2
B1   | 52   MSS_QSPI_3   B1
D1   | 53   MSS_QSPI_CLK   D1
C1   | 54   MSS_QSPI_CS   C1
K15   | 55   MSS_RGMII_RCLK   K15
G13   | 56   MSS_RGMII_RCTL   G13
M13   | 57   MSS_RGMII_RD0   M13
L15   | 58   MSS_RGMII_RD1   L15
L14   | 59   MSS_RGMII_RD2   L14
J13   | 60   MSS_RGMII_RD3   J13
H15   | 61   MSS_RGMII_TCLK   H15
G15   | 62   MSS_RGMII_TCTL   G15
J14   | 63   MSS_RGMII_TD0   J14
J15   | 64   MSS_RGMII_TD1   J15
H13   | 65   MSS_RGMII_TD2   H13
H14   | 66   MSS_RGMII_TD3   H14
R3   | 67   MSS_UARTA_RX   R3
R4   | 68   MSS_UARTA_TX   R4
P4   | 69   MSS_UARTB_TX   P4
H2   | 70   NERROR_IN   H2
H1   | 71   NERROR_OUT   H1
J3   | 72   NRESET   J3
R2   | 73   OSC_CLK_OUT_AUDIO   R2
E14   | 74   RCSS_ECAPA_CAPIN_PWMO   E14
R14   | 75   RCSS_GPIO_39   R14
R13   | 76   RCSS_I2CA_SCL   R13
P13   | 77   RCSS_I2CA_SDA   P13
B12   | 78   RCSS_MCASPA_ACLKR   B12
A12   | 79   RCSS_MCASPA_ACLKX   A12
A13   | 80   RCSS_MCASPA_AHCLKX   A13
B11   | 81   RCSS_MCASPA_DAT0   B11
C11   | 82   RCSS_MCASPA_DAT1   C11
B7   | 83   RCSS_MCASPA_DAT2   B7
C7   | 84   RCSS_MCASPA_DAT3   C7
B6   | 85   RCSS_MCASPA_DAT4   B6
A6   | 86   RCSS_MCASPA_DAT5   A6
B5   | 87   RCSS_MCASPA_DAT6   B5
A5   | 88   RCSS_MCASPA_DAT7   A5
B10   | 89   RCSS_MCASPA_DAT8   B10
A10   | 90   RCSS_MCASPA_DAT9   A10
A9   | 91   RCSS_MCASPA_DAT10   A9
C9   | 92   RCSS_MCASPA_DAT11   C9
B9   | 93   RCSS_MCASPA_DAT12   B9
A8   | 94   RCSS_MCASPA_DAT13   A8
B8   | 95   RCSS_MCASPA_DAT14   B8
A7   | 96   RCSS_MCASPA_DAT15   A7
A11   | 97   RCSS_MCASPA_FSR   A11
C12   | 98   RCSS_MCASPA_FSX   C12
P7   | 99   RCSS_MCASPB_ACLKR   P7
R8   | 100   RCSS_MCASPB_ACLKX   R8
R7   | 101   RCSS_MCASPB_AHCLKX   R7
R6   | 102   RCSS_MCASPB_DAT0   R6
N5   | 103   RCSS_MCASPB_DAT1   N5
P5   | 104   RCSS_MCASPB_DAT2   P5
R5   | 105   RCSS_MCASPB_DAT3   R5
N4   | 106   RCSS_MCASPB_DAT4   N4
N6   | 107   RCSS_MCASPB_DAT5   N6
P6   | 108   RCSS_MCASPB_FSR   P6
P8   | 109   RCSS_MCASPB_FSX   P8
R10   | 110   RCSS_MCASPC_ACLKR   R10
R9   | 111   RCSS_MCASPC_ACLKX   R9
P9   | 112   RCSS_MCASPC_AHCLKX   P9
R11   | 113   RCSS_MCASPC_DAT0   R11
P11   | 114   RCSS_MCASPC_DAT1   P11
N11   | 115   RCSS_MCASPC_DAT2   N11
R12   | 116   RCSS_MCASPC_DAT3   R12
P12   | 117   RCSS_MCASPC_DAT4   P12
N12   | 118   RCSS_MCASPC_DAT5   N12
P10   | 119   RCSS_MCASPC_FSR   P10
N9   | 120   RCSS_MCASPC_FSX   N9
P15   | 121   RCSS_MIBSPIA_CLK   P15
P14   | 122   RCSS_MIBSPIA_CS0   P14
N13   | 123   RCSS_MIBSPIA_CS1   N13
N14   | 124   RCSS_MIBSPIA_MISO   N14
N15   | 125   RCSS_MIBSPIA_MOSI   N15
E13   | 126   RCSS_UARTA_CTS   E13
F15   | 127   RCSS_UARTA_RTS   F15
G14   | 128   RCSS_UARTA_RX   G14
F14   | 129   RCSS_UARTA_TX   F14
D4   | 130   TCK   D4
C5   | 131   TDI   C5
C6   | 132   TDO   C6
L3   | 133   TEMP_SENSOR_1   L3
K3   | 134   TEMP_SENSOR_2   K3
C4   | 135   TMS   C4
H3   | 136   WARM_RESET   H3
G1   | 137   XREF_CLK0   G1
G2   | 138   XREF_CLK1   G2
[Model Data]
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[End Model Data]
[End Package Model]
| Models and submodels in the file (48): BC40D_H_PUPDOFF_5P_SC1_1P8 (I/O), BC40D_H_PD_ON_5P_!SC1_1P8 (I/O), BC40D_H_PD_ON_5P_SC1_1P8 (I/O), BC40D_H_PU_ON_5P_!SC1_1P8 (I/O), BC40D_H_PUPDOFF_5P_!SC1_1P8 (I/O), BC40D_H_PU_ON_5P_SC1_1P8 (I/O), BC40D_H_PUPDOFF_5P_SC1_3P3 (I/O), BC40D_H_PD_ON_5P_!SC1_3P3 (I/O), BC40D_H_PD_ON_5P_SC1_3P3 (I/O), BC40D_H_PU_ON_5P_!SC1_3P3 (I/O), BC40D_H_PUPDOFF_5P_!SC1_3P3 (I/O), BC40D_H_PU_ON_5P_SC1_3P3 (I/O), BC40D_H_PUPDOFF_10P_SC1_1P8 (I/O), BC40D_H_PD_ON_10P_!SC1_1P8 (I/O), BC40D_H_PD_ON_10P_SC1_1P8 (I/O), BC40D_H_PU_ON_10P_!SC1_1P8 (I/O), BC40D_H_PUPDOFF_10P_!SC1_1P8 (I/O), BC40D_H_PU_ON_10P_SC1_1P8 (I/O), BC40D_H_PUPDOFF_10P_SC1_3P3 (I/O), BC40D_H_PD_ON_10P_!SC1_3P3 (I/O), BC40D_H_PD_ON_10P_SC1_3P3 (I/O), BC40D_H_PU_ON_10P_!SC1_3P3 (I/O), BC40D_H_PUPDOFF_10P_!SC1_3P3 (I/O), BC40D_H_PU_ON_10P_SC1_3P3 (I/O), BC40D_V_PUPDOFF_5P_SC1_1P8 (I/O), BC40D_V_PD_ON_5P_!SC1_1P8 (I/O), BC40D_V_PD_ON_5P_SC1_1P8 (I/O), BC40D_V_PU_ON_5P_!SC1_1P8 (I/O), BC40D_V_PUPDOFF_5P_!SC1_1P8 (I/O), BC40D_V_PU_ON_5P_SC1_1P8 (I/O), BC40D_V_PUPDOFF_5P_SC1_3P3 (I/O), BC40D_V_PD_ON_5P_!SC1_3P3 (I/O), BC40D_V_PD_ON_5P_SC1_3P3 (I/O), BC40D_V_PU_ON_5P_!SC1_3P3 (I/O), BC40D_V_PUPDOFF_5P_!SC1_3P3 (I/O), BC40D_V_PU_ON_5P_SC1_3P3 (I/O), BC40D_V_PUPDOFF_10P_SC1_1P8 (I/O), BC40D_V_PD_ON_10P_!SC1_1P8 (I/O), BC40D_V_PD_ON_10P_SC1_1P8 (I/O), BC40D_V_PU_ON_10P_!SC1_1P8 (I/O), BC40D_V_PUPDOFF_10P_!SC1_1P8 (I/O), BC40D_V_PU_ON_10P_SC1_1P8 (I/O), BC40D_V_PUPDOFF_10P_SC1_3P3 (I/O), BC40D_V_PD_ON_10P_!SC1_3P3 (I/O), BC40D_V_PD_ON_10P_SC1_3P3 (I/O), BC40D_V_PU_ON_10P_!SC1_3P3 (I/O), BC40D_V_PUPDOFF_10P_!SC1_3P3 (I/O), BC40D_V_PU_ON_10P_SC1_3P3 (I/O)
